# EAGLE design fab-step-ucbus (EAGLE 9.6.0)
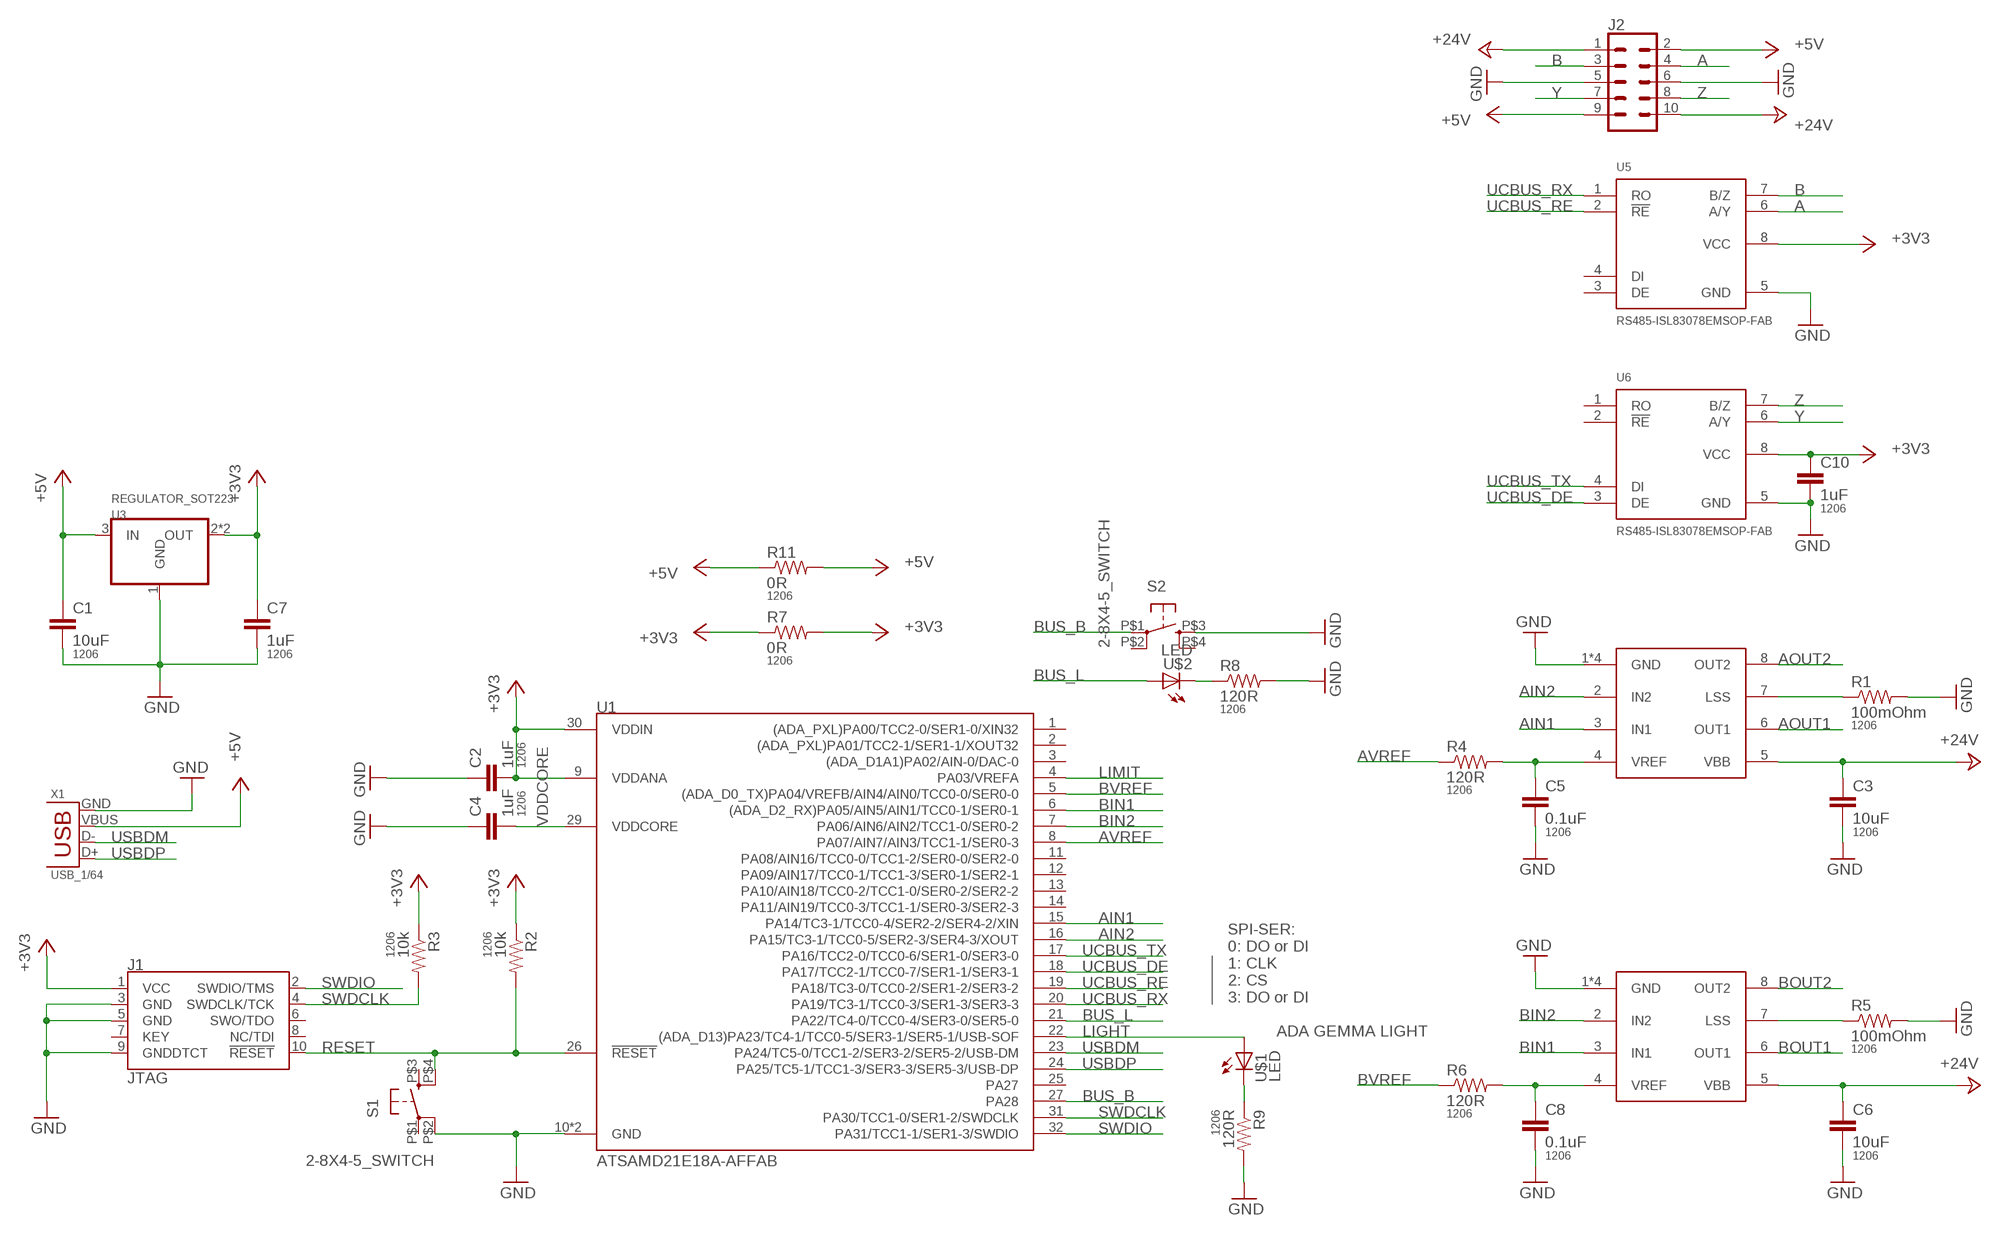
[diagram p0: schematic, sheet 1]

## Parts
C1  10uF  CAP1206  [1206]
C2  1uF  CAP1206  [1206]
C3  10uF  CAP1206  [1206]
C4  1uF  CAP1206  [1206]
C5  0.1uF  CAP1206  [1206]
C6  10uF  CAP1206  [1206]
C7  1uF  CAP1206  [1206]
C8  0.1uF  CAP1206  [1206]
C10  1uF  CAP1206  [1206]
J1  JTAG  CORTEX_JTAG_DEBUG_SMD  [2X5-SMD-1.27MM]
J2  CONN_05X2SMD_LONGPADS  [2X5-SHROUDED_SMD_LONGPADS]
R1  100mOhm  RESISTOR1206  [1206]
R2  10k  RESISTOR1206  [1206]
R3  10k  RESISTOR1206  [1206]
R4  120R  RESISTOR1206  [1206]
R5  100mOhm  RESISTOR1206  [1206]
R6  120R  RESISTOR1206  [1206]
R7  0R  RESISTOR1206  [1206]
R8  120R  RESISTOR1206  [1206]
R9  120R  RESISTOR1206  [1206]
R11  0R  RESISTOR1206  [1206]
S1  2-8X4-5_SWITCH  [TACT-SWITCH-KMR6]
S2  2-8X4-5_SWITCH  [TACT-SWITCH-KMR6]
U1  ATSAMD21E18A-AFFAB  [TQFP-32-FAB]
U2  A4950FAB  [SOIC8_PAD_THRU_FAB]
U3  REGULATOR_SOT223  [SOT223]
U4  A4950FAB  [SOIC8_PAD_THRU_FAB]
U5  RS485-ISL83078EMSOP-FAB  [8-MSOP-FAB]
U6  RS485-ISL83078EMSOP-FAB  [8-MSOP-FAB]
U$1  LED  [LED1206]
U$2  LED  [LED1206]
X1  USB_1/64  [DX4R005HJ5_64]

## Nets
+3V3: C2.2 C7.1 C10.1 J1.1(VCC) R2.1 R3.1 R7.1 R7.2 U1.9(VDDANA) U1.30(VDDIN) U3.2(OUT) U3.4(OUT) U5.8(VCC) U6.8(VCC)
+5V: C1.1 J2.2 J2.9 R11.1 R11.2 U3.3(IN) X1.VBUS
+24V: C3.1 C6.1 J2.1 J2.10 U2.5(VBB) U4.5(VBB)
A: J2.4 U5.6(A/Y)
AIN1: U1.15(PA14/TC3-1/TCC0-4/SER2-2/SER4-2/XIN) U2.3(IN1)
AIN2: U1.16(PA15/TC3-1/TCC0-5/SER2-3/SER4-3/XOUT) U2.2(IN2)
AOUT1: U2.6(OUT1)
AOUT2: U2.8(OUT2)
AVREF: R4.1 U1.8(PA07/AIN7/AIN3/TCC1-1/SER0-3)
B: J2.3 U5.7(B/Z)
BIN1: U1.6((ADA_D2_RX)PA05/AIN5/AIN1/TCC0-1/SER0-1) U4.3(IN1)
BIN2: U1.7(PA06/AIN6/AIN2/TCC1-0/SER0-2) U4.2(IN2)
BOUT1: U4.6(OUT1)
BOUT2: U4.8(OUT2)
BUS_B: S2.P$1(P) U1.27(PA28)
BUS_L: U1.21(PA22/TC4-0/TCC0-4/SER3-0/SER5-0) U$2.1(A)
BVREF: R6.1 U1.5((ADA_D0_TX)PA04/VREFB/AIN4/AIN0/TCC0-0/SER0-0)
GND: C1.2 C2.1 C3.2 C4.1 C5.2 C6.2 C7.2 C8.2 C10.2 J1.3(GND) J1.5(GND) J1.9(GNDDTCT) J2.5 J2.6 R1.2 R5.2 R8.2 R9.2 S1.P$2(P1) S2.P$3(S) U1.10(GND) U1.28(GND) U2.1(GND) U2.P$1(GND) U2.P$2(GND) U2.P$3(GND) U3.1(GND) U4.1(GND) U4.P$1(GND) U4.P$2(GND) U4.P$3(GND) U5.5(GND) U6.5(GND) X1.GND
LIGHT: U1.22((ADA_D13)PA23/TC4-1/TCC0-5/SER3-1/SER5-1/USB-SOF) U$1.1(A)
LIMIT: U1.4(PA03/VREFA)
N$1: R8.1 U$2.2(C)
N$2: R1.1 U2.7(LSS)
N$3: C5.1 R4.2 U2.4(VREF)
N$4: R5.1 U4.7(LSS)
N$5: C8.1 R6.2 U4.4(VREF)
N$6: R9.1 U$1.2(C)
RESET: J1.10(!RESET) R2.2 S1.P$4(S1) U1.26(!RESET)
SWDCLK: J1.4(SWDCLK/TCK) R3.2 U1.31(PA30/TCC1-0/SER1-2/SWDCLK)
SWDIO: J1.2(SWDIO/TMS) U1.32(PA31/TCC1-1/SER1-3/SWDIO)
UCBUS_DE: U1.18(PA17/TCC2-1/TCC0-7/SER1-1/SER3-1) U6.3(DE)
UCBUS_RE: U1.19(PA18/TC3-0/TCC0-2/SER1-2/SER3-2) U5.2(!RE)
UCBUS_RX: U1.20(PA19/TC3-1/TCC0-3/SER1-3/SER3-3) U5.1(RO)
UCBUS_TX: U1.17(PA16/TCC2-0/TCC0-6/SER1-0/SER3-0) U6.4(DI)
USBDM: U1.23(PA24/TC5-0/TCC1-2/SER3-2/SER5-2/USB-DM) X1.D-
USBDP: U1.24(PA25/TC5-1/TCC1-3/SER3-3/SER5-3/USB-DP) X1.D+
VDDCORE: C4.2 U1.29(VDDCORE)
Y: J2.7 U6.6(A/Y)
Z: J2.8 U6.7(B/Z)
Unconnected: J1.6(SWO/TDO) J1.7(KEY) J1.8(NC/TDI) S1.P$1(P) S1.P$3(S) S2.P$2(P1) S2.P$4(S1) U1.1((ADA_PXL)PA00/TCC2-0/SER1-0/XIN32) U1.2((ADA_PXL)PA01/TCC2-1/SER1-1/XOUT32) U1.3((ADA_D1A1)PA02/AIN-0/DAC-0) U1.11(PA08/AIN16/TCC0-0/TCC1-2/SER0-0/SER2-0) U1.12(PA09/AIN17/TCC0-1/TCC1-3/SER0-1/SER2-1) U1.13(PA10/AIN18/TCC0-2/TCC1-0/SER0-2/SER2-2) U1.14(PA11/AIN19/TCC0-3/TCC1-1/SER0-3/SER2-3) U1.25(PA27) U5.3(DE) U5.4(DI) U6.1(RO) U6.2(!RE)

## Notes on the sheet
- SPI-SER:
  0: DO or DI
  1: CLK
  2: CS
  3: DO or DI
- ADA GEMMA LIGHT

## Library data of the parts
C1-C8 C10 = passives:CAP: Capacitor; PACKAGE: 1206
J1 = SparkFun-Connectors:CORTEX_JTAG_DEBUG: Cortex Debug Connector - 10 pin Supports JTAG debug, Serial Wire debug, and Serial Wire Viewer. PTH and SMD connector options available. General Connector Information Products: PTH Connector -via Digi-Key SparkFun PSoc SparkFun T; PROD_ID: CONN-14503
J2 = SparkFun-Connectors:CONN_05X2: Multi connection point. Often used as Generic Header-pin footprint for 0.1 inch spaced/style header connections For AVR SPI programming port, see special device with nice symbol: "AVR_SPI_PROG_5x2.dev" You can populate with any combo of single row headers, but if you'd like an exact match, check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
R1-R9 R11 = passives:RESISTOR: Resistor; PACKAGE: 1206
S1 S2 = passives:2-8X4-5_SWITCH
U1 = microcontrollers:ATSAMD21E18A-AF: The SAM D21 is a series of low-power microcontrollers using the 32-bit ARM® Cortex® -M0+ processor, and ranging from 32- to 64-pins with up to 256KB Flash and 32KB of SRAM. The SAM D21 operate at a maximum frequency of 48MHz and reach 2.46 CoreMark® /MHz. Check prices
U2 U4 = power:A4950
U3 = power:REGULATOR_SOT223
U5 U6 = comm:RS485-ISL83078E
U$1 U$2 = fablab:LED: LED
X1 = connector:USB: SMD micro USB connector as found in the fablab inventory. Three footprint variants included: 609-4613-1-ND used by Jake original, as described by manufacturer's datasheet for milling with the 1/100" bit for milling with the 1/64" bit Made by Zaerc.

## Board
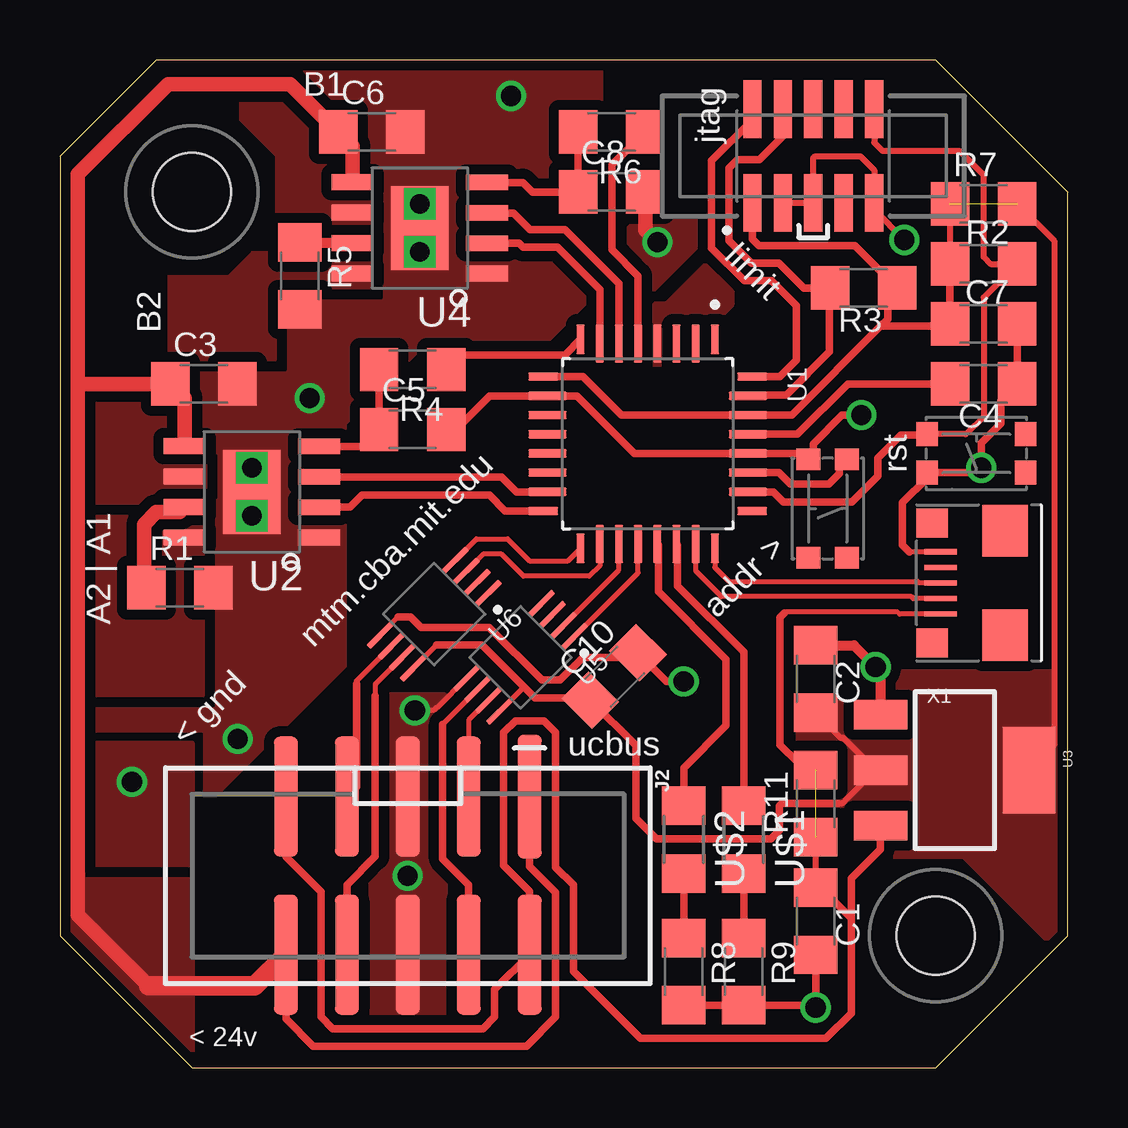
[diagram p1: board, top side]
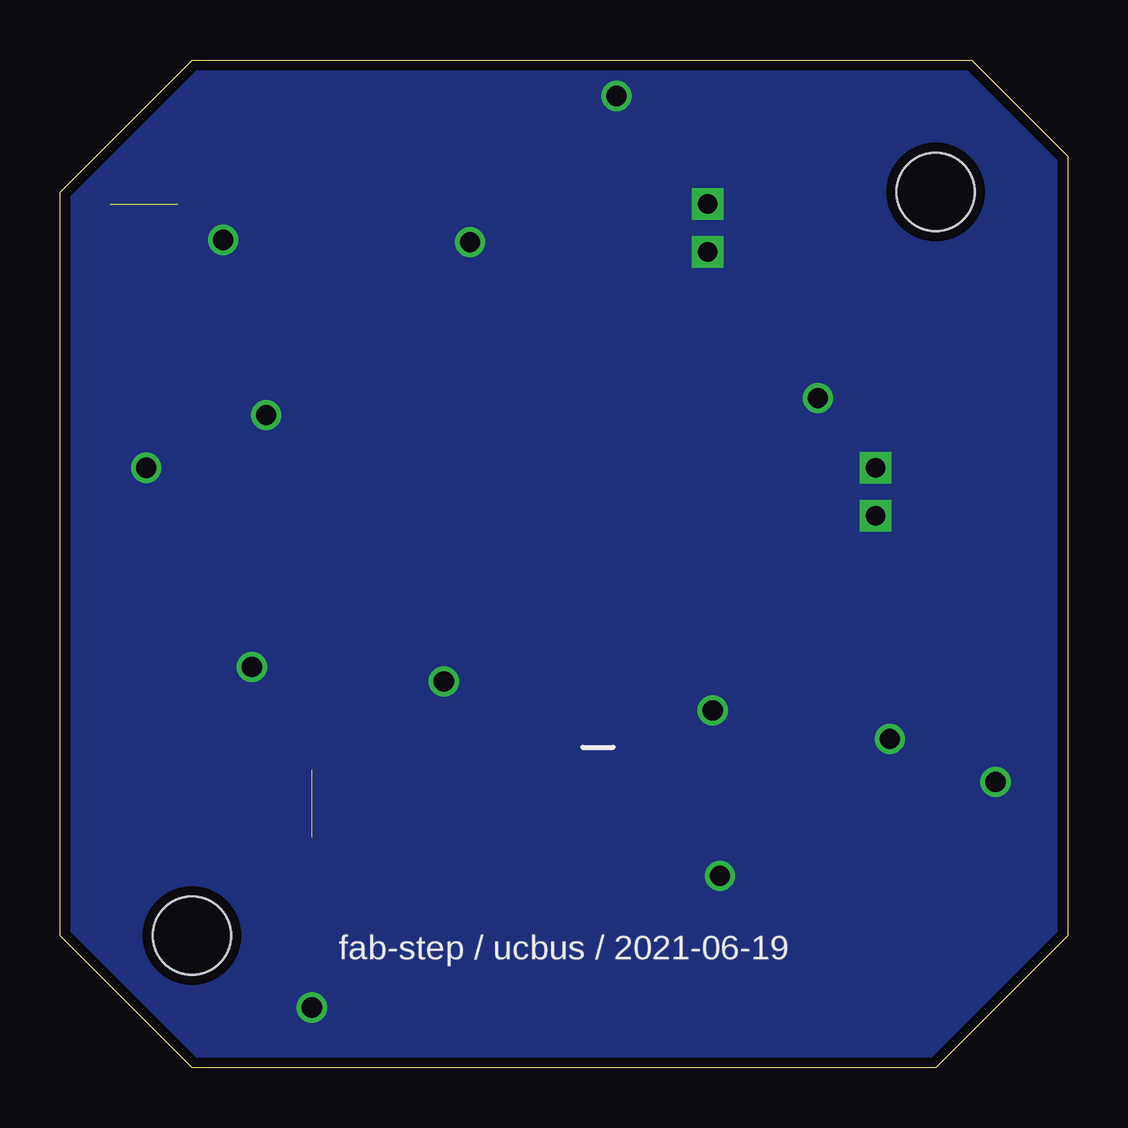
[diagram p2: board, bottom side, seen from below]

Size 42 x 42 mm. Coordinates in mm from the lower left corner, seen from the top.
Outline: 5.5,0 36.5,0 42,5.5 42,36.5 36.5,42 4,42 0,38 0,5.5 5.5,0
Copper layers (1*16): Top 0.035mm / dielectric 1.5mm / Bottom 0.035mm
Design rules "default *": minimum track width 8mil, minimum drill 33mil, track to track 17mil, track to pad 17mil, pad to pad 17mil, via to via 17mil, smd to smd 6mil, copper to edge 17mil, drill to drill 6mil, minimum pad ring 10mil, minimum via ring 8mil, stop-mask expansion 4mil, vias tented up to drill 35mil, thermal gap 17mil
Holes 3.25 mm at 36.5,5.5 5.5,36.5

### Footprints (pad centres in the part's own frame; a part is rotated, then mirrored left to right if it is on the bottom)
1206 = smd 1.6 x 1.8: 1 -1.4,0; 2 1.4,0
2X5-SMD-1.27MM = smd 0.76 x 2.4: 1 2.54,1.95; 2 2.54,-1.95; 3 1.27,1.95; 4 1.27,-1.95; 5 0,1.95; 6 0,-1.95; 7 -1.27,1.95; 8 -1.27,-1.95; 9 -2.54,1.95; 10 -2.54,-1.95
2X5-SHROUDED_SMD_LONGPADS = smd 5.15 x 1: 1 -3.294,5.08 | smd 5 x 1: 2 3.294,5.08; 3 -3.294,2.54; 4 3.294,2.54; 5 -3.294,0; 6 3.294,0; 7 -3.294,-2.54; 8 3.294,-2.54; 9 -3.294,-5.08; 10 3.294,-5.08
TACT-SWITCH-KMR6 = smd 0.9 x 1: P$1 -2.05,0.8; P$2 2.05,0.8; P$3 -2.05,-0.8; P$4 2.05,-0.8
TQFP-32-FAB = smd 1.25 x 0.35: 1 -4.355,2.8; 8 -4.355,-2.8; 17 4.355,-2.8; 24 4.355,2.8 | smd 1.6 x 0.35: 2 -4.18,2; 3 -4.18,1.2; 4 -4.18,0.4; 5 -4.18,-0.4; 6 -4.18,-1.2; 7 -4.18,-2; 18 4.18,-2; 19 4.18,-1.2; 20 4.18,-0.4; 21 4.18,0.4; 22 4.18,1.2; 23 4.18,2 | smd 0.35 x 1.25: 9 -2.8,-4.355; 16 2.8,-4.355; 25 2.8,4.355; 32 -2.8,4.355 | smd 0.35 x 1.6: 10 -2,-4.18; 11 -1.2,-4.18; 12 -0.4,-4.18; 13 0.4,-4.18; 14 1.2,-4.18; 15 2,-4.18; 26 2,4.18; 27 1.2,4.18; 28 0.4,4.18; 29 -0.4,4.18; 30 -1.2,4.18; 31 -2,4.18
SOIC8_PAD_THRU_FAB = smd 1.75 x 0.65: 1 -2.8,1.905; 2 -2.8,0.645; 3 -2.8,-0.625; 4 -2.8,-1.895; 5 2.8,-1.905; 6 2.8,-0.635; 7 2.8,0.635; 8 2.8,1.905 | smd 2.41 x 3.5: P$1 0,0 | drill 0.8 square: P$2 0,1; P$3 0,-1
SOT223 = smd 1.219 x 2.235: 1 -2.311,-3.099; 2 0,-3.099; 3 2.311,-3.099 | smd 3.6 x 2.2: 4 0,3.099
8-MSOP-FAB = smd 1.4 x 0.22: 1 -2.2,0.975; 2 -2.2,0.325; 3 -2.2,-0.325; 4 -2.2,-0.975; 5 2.2,-0.975; 6 2.2,-0.325; 7 2.2,0.325; 8 2.2,0.975
LED1206 = smd 1.6 x 1.803: 1 -1.422,0; 2 1.422,0
DX4R005HJ5_64 = smd 0.21 x 1.35: D+ 0,1.6; D- -0.65,1.6; GND 1.3,1.6; ID 0.65,1.6; VBUS -1.3,1.6 | smd 1.2 x 1.3: GND@1 -2.5,1.95; GND@2 2.5,1.95 | smd 2.15 x 1.9: GND@3 -2.175,-1.1; GND@4 2.175,-1.1

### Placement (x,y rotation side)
C1  31.5,6.1 270 top
C2  31.5,16.2 270 top
C3  6,28.5 0 top
C4  38.5,28.5 180 top
C5  14.7,26.6 0 top
C6  13,39 0 top
C7  38.5,31 0 top
C8  23,36.5 0 top
C10  23.1,16.3 45 top
J1  31.4,38 180 top
J2  14.5,8 270 top
R1  5,20 0 top
R2  38.5,33.5 0 top
R3  33.5,32.5 180 top
R4  14.7,29.1 180 top
R5  10,33 270 top
R6  23,39 180 top
R7  38.5,36 0 top
R8  26,4 270 top
R9  28.5,4 270 top
R11  31.5,11 90 top
S1  38.2,25.6 180 top
S2  32,23.3 270 top
U1  24.5,26 270 top
U2  8,24 180 top
U3  37.3,12.4 270 top
U4  15,35 180 top
U5  19.2,17.1 225 top
U6  15.6,18.9 225 top
U$1  28.5,9.5 270 top
U$2  26,9.5 270 top
X1  38.3,20.2 90 top

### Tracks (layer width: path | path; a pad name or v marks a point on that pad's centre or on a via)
+3V3  (1 unrouted)
  Top 0.203: R3.1 35.1,32.5 | U6.8 15.69,17.61 | U5.8 19.34,15.86
  Top 0.254: R7.2 41.44,34.46 41.44,13.44 U3.4 | R7.1 R2.1 | 34,12.4 33.99,12.4 32.63,13.76 32.54,13.76 C2.2 | 34,12.4 U3.2 | 32.44,11.02 32.61,11.02 32.85,11.26 32.86,11.26 34,12.4
  Top 0.305: U1.9 21.8,28.8 23.4,27.2 U1.30 30.5,27.2 34.2,30.9 | J1.1 28.86,34.54 29.13,34.27 33.13,34.27 R3.1 | 35.4,33 R3.1 | R3.1 34.5,32.1 34.5,31.2 34.2,30.9 | 34.2,30.9 37,30.9 C7.1 R2.1 | 32.44,11.02 30.09,11.02 29.99,10.91 29.99,9.88 29.64,9.54 24.86,9.54 24,10.39 24,13.42 C10.1 22.02,15.4 19.8,15.4 19.34,15.86 | 15.69,17.61 17.59,17.61 19.34,15.86 | 19.34,15.86
  pour Top (no thermals): 31.4,15.2 33.3,15.2 34.6,16.5 42.9,16.5 42.9,4.6 41.9,4.6 37.7,8.8 30.8,8.8 30.8,14.6
+5V  (1 unrouted)
  Top 0.203: X1.VBUS 35,18.9 34.9,19 30.25,19 30.2,18.95 | 19.58,3.64 J2.2
  Top 0.254: C1.1 R11.1
  Top 0.305: C1.1 31.51,7.5 31.61,7.59 32.98,6.22 | 32.98,6.22 32.98,2.27 31.93,1.22 24.2,1.22 21.4,4.01 21.4,7.61 20.66,8.34 20.66,13.96 20.18,14.45 18.98,14.45 18.5,13.96 18.5,8.43 19.58,7.34 J2.2 18.12,3.25 18.12,2.11 17.64,1.62 11.36,1.62 10.88,2.11 10.88,7.33 9.42,8.79 J2.9 | 32.98,6.22 32.98,7.88 34.2,9.1 U3.3 | R11.2 31.18,12.72 30.76,12.72 30.02,13.46 30.02,18.76 30.2,18.95
+24V
  Top 0.305: J2.1 19.58,8.39 20.66,7.3 20.66,2.11 19.44,0.89 10.56,0.89 9.42,2.02 J2.10
  Top 0.61: 0.74,28.5 0.74,37.24 4.5,41 9.6,41 C6.1 12.2,38.4 U4.5 | 0.74,28.5 C3.1 5.2,27.9 U2.5 | 0.74,28.5 0.74,6.36 3.7,3.4
  Top 0.813: J2.10 8.11,3.4 3.7,3.4
  pour Top (rank 2): 5.5,-1 5.5,8 -1,8 -1,-1
A
  Top 0.203: U5.6 15.96,14.31
  Top 0.305: J2.4 17.04,7.61 15.96,8.7 15.96,14.31
AIN1
  Top 0.305: U2.3 18.4,24.62 19.02,24 U1.15
AIN2
  Top 0.305: U2.2 12.1,23.36 12.6,23.86 17.9,23.86 18.55,23.2 U1.16
AOUT1
  pour Top (rank 2, no thermals): 6.1,23.5 1,23.5 1,29.1 6.1,29.1
AOUT2
  pour Top (no thermals): 6,23 1,23 1,15.5 6,15.5
AVREF
  Top 0.305: U1.8 21.05,29.7 16.7,29.7 R4.1
B
  Top 0.203: U5.7 17.04,14.48 J2.3
BIN1
  Top 0.305: U4.3 18.9,35.62 19.6,34.92 21.05,34.92 23.3,32.68 U1.6
BIN2
  Top 0.305: U4.2 19.13,34.35 19.3,34.19 20.75,34.19 22.5,32.44 U1.7
BOUT1
  pour Top (no thermals): 13,35 9,35 9,38 7.5,39.5 7.5,40.5 10.5,40.5 13,38
BOUT2
  pour Top (no thermals): 13,34 8,34 7,33 4.5,33 4.5,29.5 9,29.5 9,32.5 13,32.5
BUS_B
  Top 0.305: U1.27 29.97,24.8 30.46,24.32 32.04,24.32 32.48,24.76 32.48,25.03 S2.P$1
BUS_L
  Top 0.305: U1.21 24.94,21.78 24.94,19.83 27.76,17.01 27.76,14.26 26,12.5 U$2.1
BVREF
  Top 0.305: R6.1 23.38,37.98 23.36,37.98 23.02,37.64 23.02,34.08 24.1,33 U1.5
GND  (via drill 0.84)
  Top 0.203: X1.GND 35.4,21.5 | U5.5 15.71,14.99 15.67,14.99 15.57,14.89 v14.79,14.89 | U6.5 14.1,18.78
  Top 0.254: J1.3 J1.5 31.4,37.91 31.47,37.98 33.37,37.98 33.94,37.41 J1.9 33.94,35.76 v35.2,34.5
  Top 0.305: v33.4,27.2 32.6,27.2 31.4,26 31.4,25.55 S2.P$3 31,25.35 30.75,25.6 U1.28 23.96,25.6 21.56,28 U1.10 17.9,28 16.5,26.6 C5.2 | C7.2 C4.1 39.21,27.81 39.21,26.85 38.4,26.04 v38.4,25 38.2,24.8 S1.P$2 36.15,24.58 35.12,23.54 35.12,21.78 35.4,21.5 | R8.2 R9.2 31.4,2.6 v31.5,2.5 C1.2 | 14.1,18.78 14.62,18.78 15.05,18.35 17.89,18.35 20.09,16.15 20.85,16.15 21.8,17.1 23.9,17.1 C10.2 25.28,16.1 v26,16.1
  Top 0.406: U3.1 34.2,16.5 v34,16.7 33.1,17.6 C2.1
  Top 0.61: C8.2 24.4,34.9 v24.9,34.4
  other vias: 18.8,40.5 10.4,27.9 7.4,13.7 14.49,7.99 3,11.9
  pour Top (rank 6, no thermals): 22.6,42.5 22.6,32.5 20.1,30 15.1,30 11.9,26.8 11.9,16.7 6.5,11.3 6,11.3 6,14 -0.5,14 -0.5,42.5
  pour Bottom (rank 2, no thermals): -0.5,43 42.5,43 42.5,-0.5 -0.5,-0.5
  pour Top: 5.5,8.5 5.5,13.5 -1,13.5 -1,8.5
  pour Top (no thermals): 13,1.5 13,15.5 16,15.5 16,1.5
  pour Top: 24.5,32.2 26.8,34.5 26.8,35.4 24.1,35.4 23.7,35 23.7,32.8 24.3,32.2
LIGHT
  Top 0.305: U1.22 25.74,21.78 25.74,20.08 28.5,17.32 U$1.1
LIMIT
  pour Top (rank 2, no thermals): 24.6,29.3 24.6,31.6 27.05,34.05 28,33.1 28,31.8 27.5,31.3 25.8,31.3 25.2,30.7 25.2,29.3
N$1
  Top 0.305: U$2.2 R8.1
N$2
  Top 0.61: U2.7 4.99,23.16 4.02,23.16 3.5,22.64 3.5,20.1 R1.1
N$3
  Top 0.305: U2.4 12.6,25.89 C5.1 R4.2
N$4
  Top 0.406: U4.7 10.04,34.37 R5.1
N$5
  Top 0.305: U4.4 19.3,36.9 19.7,36.5 C8.1 R6.2
N$6
  Top 0.305: U$1.2 R9.1
RESET
  Top 0.254: 36.11,26.36 S1.P$4 37.75,26.4 38.5,27.15 38.5,32.1 R2.2 38.8,33.5 38.5,33.8 38.5,37.2 37.5,38.2 34.3,38.2 33.94,38.56 J1.10
  Top 0.305: 36.11,26.36 35.04,26.36 34.08,25.4 34.08,24.66 33.01,23.58 30.15,23.58 29.73,24 U1.26
SWDCLK
  Top 0.254: 32.08,32.52 R3.2
  Top 0.305: U1.31 28.72,28.04 30.28,28.04 32.08,29.84 32.08,32.52 | R3.2 31,32.5 29.97,33.53 28.83,33.53 27.9,34.46 27.9,37.49 28.24,37.83 29.15,37.83 30.13,38.81 J1.4
SWDIO
  Top 0.305: U1.32 30,28.8 30.7,29.5 30.7,31.76 29.67,32.79 28.52,32.79 27.16,34.16 27.16,37.8 28.86,39.5 J1.2
UCBUS_DE
  Top 0.203: U1.18 22.5,20.92 22.07,20.49 19.31,20.49 18.4,21.4 17.64,21.4 U6.3
UCBUS_RE
  Top 0.203: U5.2 23.3,20.74 U1.19
UCBUS_RX
  Top 0.203: U5.1 24.1,20.62 U1.20
UCBUS_TX
  Top 0.203: U6.4 17.36,22.04 18.66,22.04 19.58,21.12 21.18,21.12 U1.17
USBDM
  Top 0.203: X1.D- 35.57,19.55 35.49,19.63 27.57,19.63 26.5,20.7 U1.23
USBDP
  Top 0.203: X1.D+ 36.68,20.21 35.8,20.21 35.75,20.27 27.88,20.27 27.3,20.84 U1.24
VDDCORE
  Top 0.305: C4.2 32.84,28.5 30.74,26.4 U1.29
Y
  Top 0.203: U6.6 12.36,16.12 12.36,15.99
  Top 0.305: 12.36,15.99 12.36,11.69 J2.7
Z
  Top 0.203: U6.7 13.14,15.97 13.14,15.49
  Top 0.305: J2.8 11.96,7.61 13.14,8.8 13.14,15.49

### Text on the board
tPlace: B1 | jtag | limit | B2 | rst | mtm.cba.mit.edu | A2 | A1 | addr > | < gnd | ucbus | < 24v
bPlace: fab-step / ucbus / 2021-06-19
